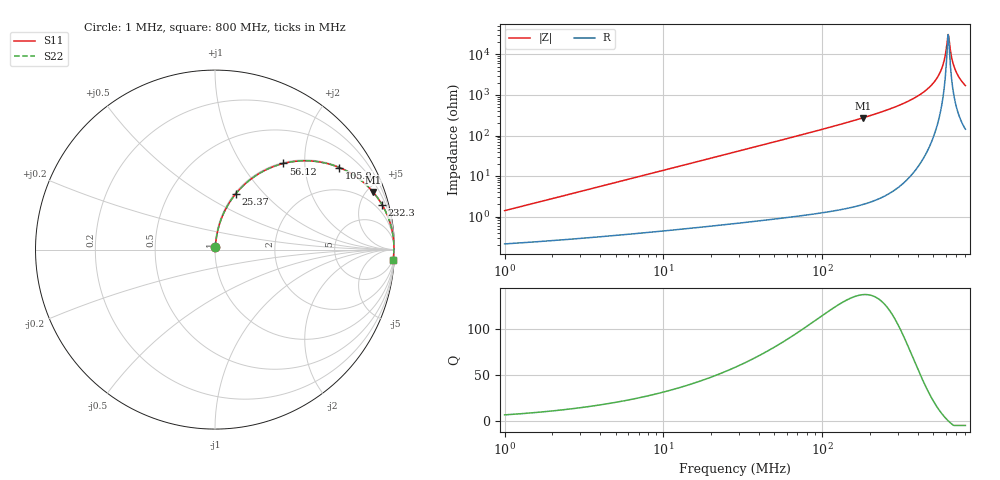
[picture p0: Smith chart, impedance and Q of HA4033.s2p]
# MHz S MA R 50
!Freq  MagS11  AngS11  MagS21  AngS21  MagS12  AngS12  MagS22  AngS22
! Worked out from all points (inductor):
!   801 points, 1 MHz to 800 MHz, reference 50 ohm
!   read as one part in series: L = 220 nH near 1.034 MHz
!   highest Q = 138 at 180.8 MHz (marker M1), where L = 240 nH
!   self-resonance near 622.6 MHz
!   S11 on the Smith chart (normalised r, x): 1 MHz: 1.00, +0.03; 25.37 MHz: 1.01, +0.70; 56.12 MHz: 1.02, +1.56; 105.9 MHz: 1.03, +3.01; 232.3 MHz: 1.06, +7.46; 800 MHz: 4, -34
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1  0.01395 80.5  0.9978 -0.8  0.9978 -0.8  0.01395 80.5
3.063851  0.04229 83.7  0.9962 -2.4  0.9962 -2.4  0.04229 83.7
9.30907  0.1272 80.8  0.9877 -7.3  0.9877 -7.3  0.1272 80.8
25.37288  0.3296 69.7  0.9381 -19.2  0.9381 -19.2  0.3296 69.7
28.28427  0.3627 67.8  0.9257 -21.3  0.9257 -21.3  0.3627 67.8
56.11923  0.6126 51.6  0.7833 -37.8  0.7833 -37.8  0.6126 51.6
86.65878  0.7703 39.1  0.6306 -50.4  0.6306 -50.4  0.7703 39.1
105.9023  0.8301 33.4  0.5507 -56.1  0.5507 -56.1  0.8301 33.4
180.7809  0.9367 20.1  0.3433 -69.5  0.3433 -69.5  0.9367 20.1
232.2835  0.964 15.0  0.2586 -74.6  0.2586 -74.6  0.964 15.0
263.3003  0.9737 12.7  0.2199 -76.8  0.2199 -76.8  0.9737 12.7
386.7043  0.9916 6.6  0.1142 -82.5  0.1142 -82.5  0.9916 6.6
492.7379  0.9962 3.2  0.05505 -84.5  0.05505 -84.5  0.9962 3.2
563.2196  0.997 1.4  0.02383 -82.1  0.02383 -82.1  0.997 1.4
587.2487  0.997 0.8  0.01428 -77.5  0.01428 -77.5  0.997 0.8
612.303  0.9969 0.2  0.005306 -54.3  0.005306 -54.3  0.9969 0.2
622.6215  0.9968 0.0  0.003195 -8.3  0.003195 -8.3  0.9968 0.0
638.4262  0.9967 -0.3  0.006265 58.0  0.006265 58.0  0.9967 -0.3
665.6639  0.9964 -0.9  0.0154 75.9  0.0154 75.9  0.9964 -0.9
694.0637  0.9959 -1.4  0.02495 79.9  0.02495 79.9  0.9959 -1.4
742.045  0.9949 -2.3  0.04042 81.7  0.04042 81.7  0.9949 -2.3
800  0.9935 -3.3  0.05804 81.9  0.05804 81.9  0.9935 -3.3
